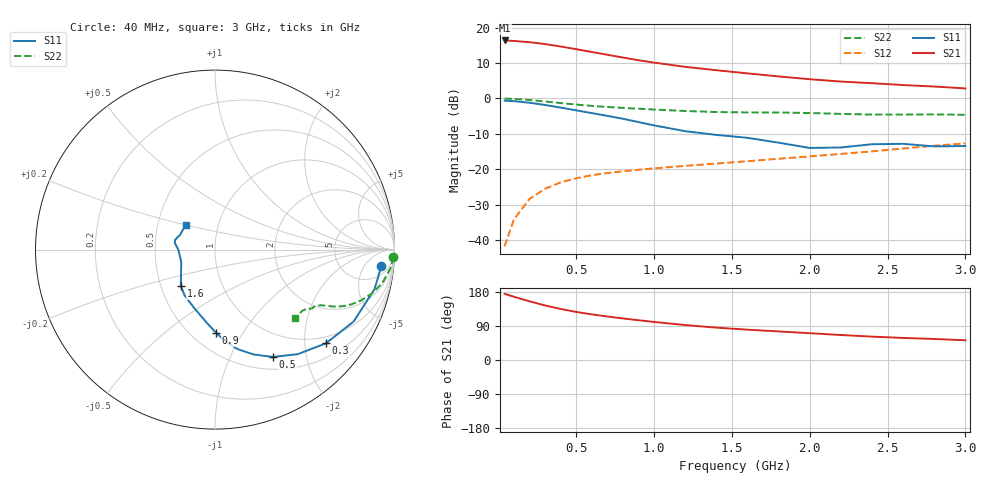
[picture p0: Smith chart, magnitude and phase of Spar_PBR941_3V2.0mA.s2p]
! Filename:  PBR941C.S2P  Version:  3.0
! NXP part #:  PBR941  Date: July 1998
! Bias condition:  Vce=3V, Ic=2.0mA
#  MHz  S  MA  R 50
! Freq  S11  S21  S12  S22
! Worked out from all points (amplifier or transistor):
!   21 points, 40 MHz to 3 GHz, reference 50 ohm
!   highest |S21| = 16.4 dB at 40 MHz (marker M1)
!   |S21| within 3 dB of that: start of sweep to 567.8 MHz
!   unconditionally stable (mu >= 1): 1.722 GHz to end of sweep
!   at 300 MHz: K = 0.27, MSG = 20.4 dB, |S12| = -25.5 dB
!   at 1 GHz: K = 0.75, MSG = 14.9 dB, |S12| = -19.7 dB
!   at 3 GHz: K = 1.02, MAG = 6.9 dB, |S12| = -12.7 dB
!   S11 on the Smith chart (normalised r, x): 40 MHz: 10, -13; 300 MHz: 0.83, -2.50; 500 MHz: 0.66, -1.46; 900 MHz: 0.65, -0.77; 1.6 GHz: 0.63, -0.28; 3 GHz: 0.69, +0.20
40  0.9315 -5.6  6.574 174.6  0.00826 86.7  0.9942 -2.4
100  0.9158 -13.9  6.474 166.9  0.0197 82.5  0.9842 -5.9
200  0.8701 -27.4  6.209 154.8  0.03836 74.9  0.9509 -11.3
300  0.8095 -40.1  5.851 144.0  0.05326 69.3  0.9064 -15.8
400  0.7429 -51.6  5.4 134.7  0.06556 64.6  0.8607 -19.2
500  0.6791 -61.7  4.953 126.8  0.07491 61.6  0.8199 -21.8
600  0.6216 -69.9  4.519 120.4  0.08279 59.6  0.7856 -23.6
700  0.569 -77.1  4.13 114.8  0.08871 58.5  0.7584 -24.7
800  0.5167 -83.3  3.775 109.7  0.09397 58.0  0.7362 -25.6
900  0.4645 -89.1  3.462 105.0  0.09879 57.9  0.7164 -26.1
1000  0.4171 -95.4  3.202 100.5  0.1034 58.2  0.6983 -26.6
1200  0.3456 -109.6  2.793 92.2  0.1122 59.3  0.6662 -27.7
1400  0.3062 -123.6  2.499 85.4  0.1209 60.9  0.6434 -29.1
1600  0.2785 -133.1  2.258 80.0  0.1302 63.3  0.6358 -30.3
1800  0.2379 -142.8  2.045 75.4  0.1411 66.2  0.6334 -31.1
2000  0.2005 -159.4  1.867 70.7  0.1522 68.2  0.6234 -31.9
2200  0.2036 -179.3  1.732 66.0  0.1651 69.9  0.6054 -33.1
2400  0.2261 170.9  1.64 61.7  0.1795 71.5  0.5923 -35.4
2600  0.2292 166.1  1.545 58.2  0.1968 73.3  0.5925 -38.0
2800  0.2109 157.1  1.473 55.5  0.2153 74.5  0.596 -39.8
3000  0.2135 140.2  1.385 52.0  0.2324 75.1  0.5875 -40.8
